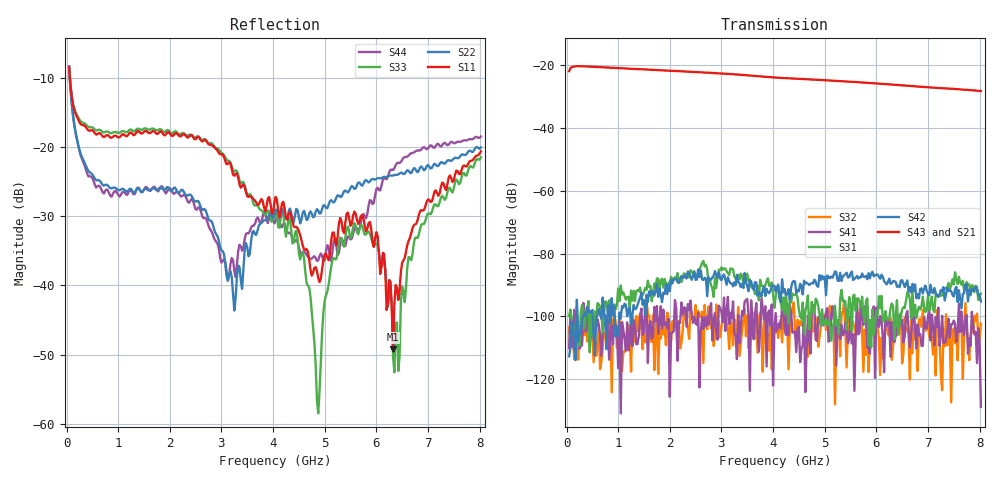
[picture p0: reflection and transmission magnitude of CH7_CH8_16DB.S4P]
!Agilent Technologies,E5071C,MY46316741,A.11.02
!Date: Mon Jun 01 10:28:31 2026
!Data & Calibration Information:
!1:CH7 INPUT 2:CH7 OUTPUT 3:CH8 INPUT 4:CH8 OUTPUT
!Freq	S11:SOLT4(ON)	S12:SOLT4(ON)	S13:SOLT4(ON)	S14:SOLT4(ON)
!	S21:SOLT4(ON)	S22:SOLT4(ON)	S23:SOLT4(ON)	S24:SOLT4(ON)
!	S31:SOLT4(ON)	S32:SOLT4(ON)	S33:SOLT4(ON)	S34:SOLT4(ON)
!	S41:SOLT4(ON)	S42:SOLT4(ON)	S43:SOLT4(ON)	S44:SOLT4(ON)
!PortZ  Port1:50+j0  Port2:50+j0  Port3:50+j0  Port4:50+j0
!Above PortZ is port z conversion or system Z0 setting when saving the data.
!When reading, reference impedance value at option line is always used.
# Hz S dB R 50
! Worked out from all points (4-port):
!   320 points, 50 MHz to 8.025 GHz, reference 50 ohm
!   strongest paths, dB at 50 MHz, 2.05 GHz, 4.05 GHz, 6.05 GHz, 8.025 GHz:
!     S43: -21.8, -21.8, -23.9, -25.8, -28.2
!     S21: -21.9, -21.8, -24.0, -26.0, -28.4
!     S42: -112.7, -89.5, -92.0, -87.3, -95.2
!     S31: -99.9, -88.1, -93.8, -93.5, -92.7
!     S41: -110.1, -105.1, -98.9, -103.3, -128.8
!     S32: -103.4, -101.5, -105.2, -106.9, -102.3
!   lowest |S11| = -49.2 dB at 6.325 GHz (marker M1), VSWR 1.01, Z = 49.7 - j0.199 ohm
!   |S11| at or under -10 dB: 64.84 MHz to end of sweep
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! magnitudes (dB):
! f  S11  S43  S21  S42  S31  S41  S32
! 50 MHz  -8.5  -21.8  -21.9  -112.7  -99.9  -110.1  -103.4
! 3.25 GHz  -24.2  -22.9  -23.0  -89.1  -87.2  -105.4  -100.8
! 4.45 GHz  -31.5  -24.3  -24.4  -92.6  -92.8  -111.3  -107.9
! 4.875 GHz  -38.9  -24.6  -24.8  -90.5  -96.7  -100.2  -109.6
! 5.45 GHz  -29.5  -25.2  -25.3  -87.5  -98.2  -108.6  -102.9
! 6.325 GHz  -49.2  -26.2  -26.4  -88.7  -96.8  -107.3  -109.2
! 8.025 GHz  -20.6  -28.2  -28.4  -95.2  -92.7  -128.8  -102.3
